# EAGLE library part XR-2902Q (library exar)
MICROCONTROLLER
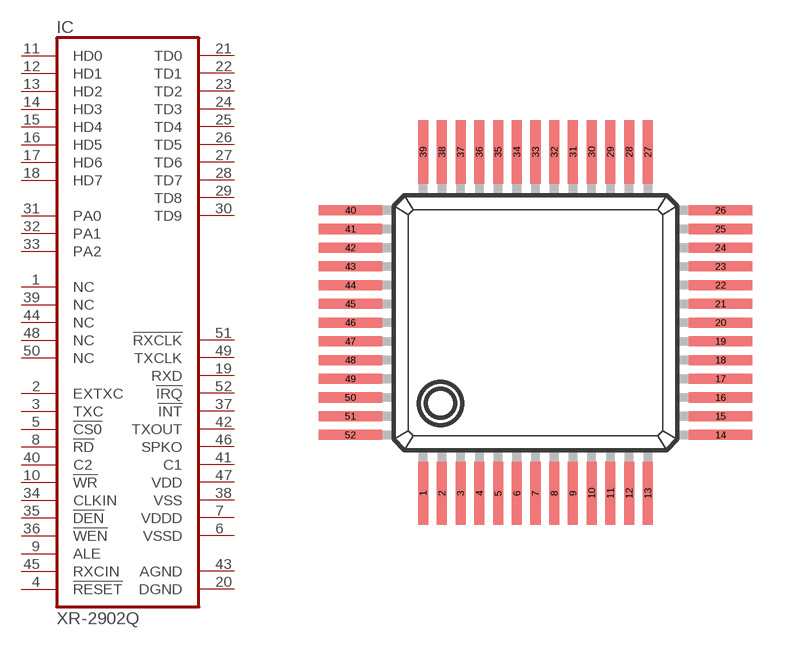
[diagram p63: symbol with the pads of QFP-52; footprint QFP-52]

Designator prefix IC

## XR-2902Q (OC_FARNELL: unknown; OC_NEWARK: unknown)  [QFP-52]
1  NC  nc
2  EXTXC  in
3  TXC  in
4  !RESET  in
5  !CS0  in
6  VSSD  pwr
7  VDDD  pwr
8  !RD  in
9  ALE  in
10  !WR  in
11  HD0
12  HD1
13  HD2
14  HD3
15  HD4
16  HD5
17  HD6
18  HD7
19  RXD  out
20  DGND  pwr
21  TD0
22  TD1
23  TD2
24  TD3
25  TD4
26  TD5
27  TD6
28  TD7
29  TD8
30  TD9
31  PA0
32  PA1
33  PA2
34  CLKIN  in
35  !DEN  in
36  !WEN  in
37  !INT  out
38  VSS  pwr
39  NC  nc
40  C2  in
41  C1  out
42  TXOUT  out
43  AGND  pwr
44  NC  nc
45  RXCIN  in
46  SPKO  out
47  VDD  pwr
48  NC  nc
49  TXCLK  out
50  NC  nc
51  !RXCLK  out
52  !IRQ  out

## Footprint QFP-52 (pad centres in mm)
Quad Flat Package
smd 0.35 x 2.2: 1 -3.575,-6.25; 2 -2.925,-6.25; 3 -2.275,-6.25; 4 -1.625,-6.25; 5 -0.975,-6.25; 6 -0.325,-6.25; 7 0.325,-6.25; 8 0.975,-6.25; 9 1.625,-6.25; 10 2.275,-6.25; 11 2.925,-6.25; 12 3.575,-6.25; 13 4.225,-6.25; 27 4.225,5.6; 28 3.575,5.6; 29 2.925,5.6; 30 2.275,5.6; 31 1.625,5.6; 32 0.975,5.6; 33 0.325,5.6; 34 -0.325,5.6; 35 -0.975,5.6; 36 -1.625,5.6; 37 -2.275,5.6; 38 -2.925,5.6; 39 -3.575,5.6
smd 2.2 x 0.35: 14 6.75,-4.225; 15 6.75,-3.575; 16 6.75,-2.925; 17 6.75,-2.275; 18 6.75,-1.625; 19 6.75,-0.975; 20 6.75,-0.325; 21 6.75,0.325; 22 6.75,0.975; 23 6.75,1.625; 24 6.75,2.275; 25 6.75,2.925; 26 6.75,3.575; 40 -6.1,3.575; 41 -6.1,2.925; 42 -6.1,2.275; 43 -6.1,1.625; 44 -6.1,0.975; 45 -6.1,0.325; 46 -6.1,-0.325; 47 -6.1,-0.975; 48 -6.1,-1.625; 49 -6.1,-2.275; 50 -6.1,-2.925; 51 -6.1,-3.575; 52 -6.1,-4.225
